| IBIS file stm32f413_f423_ufbga144.ibs
[IBIS ver] 4.2
[File name] stm32f413_f423_ufbga144.ibs
[File Rev] 1.2
[Date]  18-05-2020
[Source] Data Created at STMicroelectronics
[Notes]  File originated from ELDO simulations. rev 1.1: removal of the rising/falling waveform I2C
[Disclaimer]  This information is for modeling purpose only and is
   not guaranted. The information is subject to change without
   notice.
[Copyright] Copyright 2020 STMicroelectronics Inc.
|   Component stm32f413_f423_ufbga144
[Component] stm32f413_f423_ufbga144
[Manufacturer] STMicroelectronics
[Package]
| variable   typ   min   max
R_pkg   0.0   0.0   0.0
L_pkg   0.0H   0.0H   0.0H
C_pkg   0.0F   0.0F   0.0F
[Pin]  signal_name   model_name   R_pin   L_pin   C_pin
A1 PC13-ANTI_TAMP io8p_arwsudq_ft_v33
A10 PA15 io8p_arsudq_ft
A11 PA14 io8p_arsudq_ft
A12 PA13 io8p_arsudq_ft
A2 PE3 io8p_arsudq_ft
A3 PE2 io8p_arsudq_ft
A4 PE1 io8p_arsudq_ft
A5 PE0 io8p_arsudq_ft
A6 PB4 io8p_arsudq_i2cin_ft
A7 PB3 io8p_arsudq_i2c_ft
A8 PD6 io8p_arsudq_ft
A9 PD7 io8p_arsudq_ft
B1 PC14-OSC32_IN io8p_arwsudq_ft
B10 PC11 io8p_arsudq_ft
B11 PC10 io8p_arsudq_ft
B12 PA12 io8usb_vbus_otg_ft
B2 PE4 io8p_arsudq_ft
B3 PE5 io8p_arsudq_ft
B4 PE6 io8p_arsudq_ft
B5 PB9 io8p_arsudq_i2cin_ft
B6 PB5 io8p_ar3wsudq_ft
B7 PG15 io8p_arsudq_ft
B8 PG12 io8p_arsudq_ft
B9 PD5 io8p_arsudq_ft
C1 PC15-OSC32_OUT io8p_arsudq_ft
C10 PC12 io8p_arsudq_ft
C11 VDD_2_USB33 POWER
C12 PA11 io8usb_lsfs_otg_ft
C2 VBAT POWER
C3 PF0 io8p_arsudq_i2cin_ft
C4 PF1 io8p_arsudq_i2cin_ft
C5 PB8 io8p_arsudq_i2cin_ft
C6 PB6 io8p_arsudq_i2cin_ft
C7 PG14 io8p_arsudq_ft
C8 PG11 io8p_arsudq_ft
C9 PD4 io8p_arsudq_ft
D1 PH0-OSC_IN io8p_arsudq_ft
D10 PD1 io8p_arsudq_ft
D11 PA10 io8usb_id_otg_ft
D12 PA9 io8usb_vbus_otg_ft
D2 VSS_5 GND
D3 VDD_5 POWER
D4 PF2 io8p_arsudq_ft
D5 BOOT0 vpp_test_hv
D6 PB7 io8p_arsudq_i2cin_ft
D7 PG13 io8p_arsudq_ft
D8 PG10 io8p_arsudq_ft
D9 PD3 io8p_arsudq_ft
E1 PH1-OSC_OUT io8p_arsudq_ft
E10 PD0 io8p_arsudq_ft
E11 PC9 io8p_arsudq_i2cin_ft
E12 PA8 io8p_arsudq_i2cin_ft
E2 PF3 io8p_arsudq_ft
E3 PF4 io8p_arsudq_ft
E4 PF5 io8p_arsudq_ft
E5 PDR_ON GND
E6 VSS_3 GND
E7 VSS_10 GND
E8 PG9 io8p_arsudq_ft
E9 PD2 io8p_arsudq_ft
F1 NRST ioreset_ft_v33
F10 VDD_9 POWER
F11 PC8 io8p_arsudq_ft
F12 PC7 io8p_arsudq_i2c_ft
F2 PF7 io8p_arsudq_ft
F3 PF6 io8p_arsudq_ft
F4 VDD_4 POWER
F5 VDD_3 POWER
F6 VDD_11 POWER
F7 VDD_10 POWER
F8 VDD_8 POWER
F9 VDD_2_0 POWER
G1 PF10 io8p_arsudq_ft
G10 VSS_2_0 GND
G11 PG8 io8p_arsudq_ft
G12 PC6 io8p_arsudq_i2c_ft
G2 PF9 io8p_arsudq_ft
G3 PF8 io8p_arsudq_ft
G4 VSS_6 GND
G5 VDD_6 POWER
G6 VDD_7 POWER
G7 VDD_1_0 POWER
G8 VSS_8 GND
G9 VCAP2_0 POWER
H1 PC0 io8p_arwsudq_ft_v33
H10 PG7 io8p_arsudq_ft
H11 PG6 io8p_arsudq_ft
H12 PG5 io8p_arsudq_ft
H2 PC1 io8p_arwsudq_ft_v33
H3 PC2 io8p_arwsudq_ft
H4 PC3 io8p_arwsudq_ft
H5 BYPASS_USER GND
H6 VSS_7 GND
H7 VCAP1_0 POWER
H8 PE11 io8p_arsudq_ft
H9 PD11 io8p_arsudq_ft
J1 VSSA GND
J10 PG4 io8p_arsudq_ft
J11 PG3 io8p_arsudq_ft
J12 PG2 io8p_arsudq_ft
J2 PA0-WKUP io8p_arwsudq_ft_v33
J3 PA4 io8p_ar3wsudq_ft
J4 PC4 io8p_arwsudq_ft
J5 PB2 io8p_arwsudq_ft
J6 PG1 io8p_arsudq_ft
J7 PE10 io8p_arsudq_ft
J8 PE12 io8p_arsudq_ft
J9 PD10 io8p_arsudq_ft
K1 VREF- GND
K10 PD13 io8p_arsudq_i2c_ft
K11 PD14 io8p_arsudq_i2c_ft
K12 PD15 io8p_arsudq_i2c_ft
K2 PA1 io8p_arwsudq_ft
K3 PA5 io8p_ar3wsudq_ft
K4 PC5 io8p_arwsudq_ft
K5 PF13 io8p_arsudq_ft
K6 PG0 io8p_arsudq_ft
K7 PE9 io8p_arsudq_ft
K8 PE13 io8p_arsudq_ft
K9 PD9 io8p_arsudq_ft
L1 VREF+ POWER
L10 PD12 io8p_arsudq_i2c_ft
L11 PB14 io8p_arsudq_i2c_ft
L12 PB15 io8p_arsudq_i2c_ft
L2 PA2 io8p_arwsudq_ft
L3 PA6 io8p_ar3wsudq_ft
L4 PB0 io8p_ar3wsudq_ft
L5 PF12 io8p_arsudq_ft
L6 PF15 io8p_arsudq_i2c_ft
L7 PE8 io8p_arsudq_ft
L8 PE14 io8p_arsudq_ft
L9 PD8 io8p_arsudq_ft
M1 VDDA POWER
M10 PB11 io8p_arsudq_i2cin_ft
M11 PB12 io8p_arsudq_ft
M12 PB13 io8p_arsudq_ft
M2 PA3 io8p_arwsudq_ft
M3 PA7 io8p_arwsudq_ft
M4 PB1 io8p_ar3wsudq_ft
M5 PF11 io8p_arsudq_ft
M6 PF14 io8p_arsudq_i2c_ft
M7 PE7 io8p_arsudq_ft
M8 PE15 io8p_ar3wsudq_ft
M9 PB10 io8p_arsudq_i2c_ft
[Model Selector] io8p_ar3wsudq_ft
io8p00_ar3wsudq_ft_pd_lv  "SPEED00 1P8V, PD=40kOhm"
io8p00_ar3wsudq_ft_pu_lv  "SPEED00 1P8V, PU=40kOhm"
io8p00_ar3wsudq_ft_lv  "SPEED00 1P8V"
io8p01_ar3wsudq_ft_pd_lv  "SPEED01 1P8V, PD=40kOhm"
io8p01_ar3wsudq_ft_pu_lv  "SPEED01 1P8V, PU=40kOhm"
io8p01_ar3wsudq_ft_lv  "SPEED01 1P8V"
io8p10_ar3wsudq_ft_pd_lv  "SPEED10 1P8V, PD=40kOhm"
io8p10_ar3wsudq_ft_pu_lv  "SPEED10 1P8V, PU=40kOhm"
io8p10_ar3wsudq_ft_lv  "SPEED10 1P8V"
io8p11_ar3wsudq_ft_pd_lv  "SPEED11 1P8V, PD=40kOhm"
io8p11_ar3wsudq_ft_pu_lv  "SPEED11 1P8V, PU=40kOhm"
io8p11_ar3wsudq_ft_lv  "SPEED11 1P8V"
io8p00_ar3wsudq_ft_pd  "SPEED00, PD=40kOhm"
io8p00_ar3wsudq_ft_pu  "SPEED00, PU=40kOhm"
io8p00_ar3wsudq_ft  "SPEED00"
io8p01_ar3wsudq_ft_pd  "SPEED01, PD=40kOhm"
io8p01_ar3wsudq_ft_pu  "SPEED01, PU=40kOhm"
io8p01_ar3wsudq_ft  "SPEED01"
io8p10_ar3wsudq_ft_pd  "SPEED10, PD=40kOhm"
io8p10_ar3wsudq_ft_pu  "SPEED10, PU=40kOhm"
io8p10_ar3wsudq_ft  "SPEED10"
io8p11_ar3wsudq_ft_pd  "SPEED11, PD=40kOhm"
io8p11_ar3wsudq_ft_pu  "SPEED11, PU=40kOhm"
io8p11_ar3wsudq_ft  "SPEED11"
[Model Selector] io8p_arsudq_ft
io8p00_arsudq_ft_pd_lv  "SPEED00 1P8V, PD=40kOhm"
io8p00_arsudq_ft_pu_lv  "SPEED00 1P8V, PU=40kOhm"
io8p00_arsudq_ft_lv  "SPEED00 1P8V"
io8p01_arsudq_ft_pd_lv  "SPEED01 1P8V, PD=40kOhm"
io8p01_arsudq_ft_pu_lv  "SPEED01 1P8V, PU=40kOhm"
io8p01_arsudq_ft_lv  "SPEED01 1P8V"
io8p10_arsudq_ft_pd_lv  "SPEED10 1P8V, PD=40kOhm"
io8p10_arsudq_ft_pu_lv  "SPEED10 1P8V, PU=40kOhm"
io8p10_arsudq_ft_lv  "SPEED10 1P8V"
io8p11_arsudq_ft_pd_lv  "SPEED11 1P8V, PD=40kOhm"
io8p11_arsudq_ft_pu_lv  "SPEED11 1P8V, PU=40kOhm"
io8p11_arsudq_ft_lv  "SPEED11 1P8V"
io8p00_arsudq_ft_pd  "SPEED00, PD=40kOhm"
io8p00_arsudq_ft_pu  "SPEED00, PU=40kOhm"
io8p00_arsudq_ft  "SPEED00"
io8p01_arsudq_ft_pd  "SPEED01, PD=40kOhm"
io8p01_arsudq_ft_pu  "SPEED01, PU=40kOhm"
io8p01_arsudq_ft  "SPEED01"
io8p10_arsudq_ft_pd  "SPEED10, PD=40kOhm"
io8p10_arsudq_ft_pu  "SPEED10, PU=40kOhm"
io8p10_arsudq_ft  "SPEED10"
io8p11_arsudq_ft_pd  "SPEED11, PD=40kOhm"
io8p11_arsudq_ft_pu  "SPEED11, PU=40kOhm"
io8p11_arsudq_ft  "SPEED11"
[Model Selector] io8p_arsudq_i2c_ft
io8prog_1v8_i2c_pd  "5V Tol GPIO 1.8V range i2c functionality with pull down"
io8prog_1v8_i2c_pu  "5V Tol GPIO 1.8V range i2c functionality with pull up"
io8prog_1v8_i2c  "5V Tol GPIO 1.8V range i2c functionality"
io8prog_3v3_i2c_pd  "5V Tol GPIO 3.3V range i2c functionality with pull down"
io8prog_3v3_i2c_pu  "5V Tol GPIO 3.3V range i2c functionality with pull up"
io8prog_3v3_i2c  "5V Tol GPIO 3.3V range i2c functionality"
io8prog_1v8_pd_00  "5V Tol GPIO 1.8V range with pd speed 00"
io8prog_1v8_pu_00  "5V Tol GPIO 1.8V range with pu speed 00"
io8prog_1v8_00  "5V Tol GPIO 1.8V range speed 00"
io8prog_3v3_pd_00  "5V Tol GPIO 3.3V range with pd speed 00"
io8prog_3v3_pu_00  "5V Tol GPIO 3.3V range with pu speed 00"
io8prog_3v3_00  "5V Tol GPIO 3.3V range speed 00"
io8prog_1v8_pd_01  "5V Tol GPIO 1.8V range with pd speed 01"
io8prog_1v8_pu_01  "5V Tol GPIO 1.8V range with pu speed 01"
io8prog_1v8_01  "5V Tol GPIO 1.8V range speed 01"
io8prog_3v3_pd_01  "5V Tol GPIO 3.3V range with pd speed 01"
io8prog_3v3_pu_01  "5V Tol GPIO 3.3V range with pu speed 01"
io8prog_3v3_01  "5V Tol GPIO 3.3V range speed 01"
io8prog_1v8_pd_10  "5V Tol GPIO 1.8V range with pd speed 10"
io8prog_1v8_pu_10  "5V Tol GPIO 1.8V range with pu speed 10"
io8prog_1v8_10  "5V Tol GPIO 1.8V range speed 10"
io8prog_3v3_pd_10  "5V Tol GPIO 3.3V range with pd speed 10"
io8prog_3v3_pu_10  "5V Tol GPIO 3.3V range with pu speed 10"
io8prog_3v3_10  "5V Tol GPIO 3.3V range speed 10"
io8prog_1v8_pd_11  "5V Tol GPIO 1.8V range with pd speed 11"
io8prog_1v8_pu_11  "5V Tol GPIO 1.8V range with pu speed 11"
io8prog_1v8_11  "5V Tol GPIO 1.8V range speed 11"
io8prog_3v3_pd_11  "5V Tol GPIO 3.3V range with pd speed 11"
io8prog_3v3_pu_11  "5V Tol GPIO 3.3V range with pu speed 11"
io8prog_3v3_11  "5V Tol GPIO 3.3V range speed 11"
[Model Selector] io8p_arsudq_i2cin_ft
io8p00_arsudq_i2cin_ft_pd_lv  "SPEED00 1P8V, PD=40kOhm"
io8p00_arsudq_i2cin_ft_pu_lv  "SPEED00 1P8V, PU=40kOhm"
io8p00_arsudq_i2cin_ft_lv  "SPEED00 1P8V"
io8p01_arsudq_i2cin_ft_pd_lv  "SPEED01 1P8V, PD=40kOhm"
io8p01_arsudq_i2cin_ft_pu_lv  "SPEED01 1P8V, PU=40kOhm"
io8p01_arsudq_i2cin_ft_lv  "SPEED01 1P8V"
io8p10_arsudq_i2cin_ft_pd_lv  "SPEED10 1P8V, PD=40kOhm"
io8p10_arsudq_i2cin_ft_pu_lv  "SPEED10 1P8V, PU=40kOhm"
io8p10_arsudq_i2cin_ft_lv  "SPEED10 1P8V"
io8p11_arsudq_i2cin_ft_pd_lv  "SPEED11 1P8V, PD=40kOhm"
io8p11_arsudq_i2cin_ft_pu_lv  "SPEED11 1P8V, PU=40kOhm"
io8p11_arsudq_i2cin_ft_lv  "SPEED11 1P8V"
io8p00_arsudq_i2cin_ft_pd  "SPEED00, PD=40kOhm"
io8p00_arsudq_i2cin_ft_pu  "SPEED00, PU=40kOhm"
io8p00_arsudq_i2cin_ft  "SPEED00"
io8p01_arsudq_i2cin_ft_pd  "SPEED01, PD=40kOhm"
io8p01_arsudq_i2cin_ft_pu  "SPEED01, PU=40kOhm"
io8p01_arsudq_i2cin_ft  "SPEED01"
io8p10_arsudq_i2cin_ft_pd  "SPEED10, PD=40kOhm"
io8p10_arsudq_i2cin_ft_pu  "SPEED10, PU=40kOhm"
io8p10_arsudq_i2cin_ft  "SPEED10"
io8p11_arsudq_i2cin_ft_pd  "SPEED11, PD=40kOhm"
io8p11_arsudq_i2cin_ft_pu  "SPEED11, PU=40kOhm"
io8p11_arsudq_i2cin_ft  "SPEED11"
[Model Selector] io8p_arwsudq_ft
io8p00_arwsudq_ft_pd_lv  "SPEED00 1P8V, PD=40kOhm"
io8p00_arwsudq_ft_pu_lv  "SPEED00 1P8V, PU=40kOhm"
io8p00_arwsudq_ft_lv  "SPEED00 1P8V"
io8p01_arwsudq_ft_pd_lv  "SPEED01 1P8V, PD=40kOhm"
io8p01_arwsudq_ft_pu_lv  "SPEED01 1P8V, PU=40kOhm"
io8p01_arwsudq_ft_lv  "SPEED01 1P8V"
io8p10_arwsudq_ft_pd_lv  "SPEED10 1P8V, PD=40kOhm"
io8p10_arwsudq_ft_pu_lv  "SPEED10 1P8V, PU=40kOhm"
io8p10_arwsudq_ft_lv  "SPEED10 1P8V"
io8p11_arwsudq_ft_pd_lv  "SPEED11 1P8V, PD=40kOhm"
io8p11_arwsudq_ft_pu_lv  "SPEED11 1P8V, PU=40kOhm"
io8p11_arwsudq_ft_lv  "SPEED11 1P8V"
io8p00_arwsudq_ft_pd  "SPEED00, PD=40kOhm"
io8p00_arwsudq_ft_pu  "SPEED00, PU=40kOhm"
io8p00_arwsudq_ft  "SPEED00"
io8p01_arwsudq_ft_pd  "SPEED01, PD=40kOhm"
io8p01_arwsudq_ft_pu  "SPEED01, PU=40kOhm"
io8p01_arwsudq_ft  "SPEED01"
io8p10_arwsudq_ft_pd  "SPEED10, PD=40kOhm"
io8p10_arwsudq_ft_pu  "SPEED10, PU=40kOhm"
io8p10_arwsudq_ft  "SPEED10"
io8p11_arwsudq_ft_pd  "SPEED11, PD=40kOhm"
io8p11_arwsudq_ft_pu  "SPEED11, PU=40kOhm"
io8p11_arwsudq_ft  "SPEED11"
[Model Selector] io8p_arwsudq_ft_v33
io8p00_arwsudq_ft_v33_pd_lv  "SPEED00 1P8V, PD=40kOhm"
io8p00_arwsudq_ft_v33_pu_lv  "SPEED00 1P8V, PU=40kOhm"
io8p00_arwsudq_ft_v33_lv  "SPEED00 1P8V"
io8p01_arwsudq_ft_v33_pd_lv  "SPEED01 1P8V, PD=40kOhm"
io8p01_arwsudq_ft_v33_pu_lv  "SPEED01 1P8V, PU=40kOhm"
io8p01_arwsudq_ft_v33_lv  "SPEED01 1P8V"
io8p10_arwsudq_ft_v33_pd_lv  "SPEED10 1P8V, PD=40kOhm"
io8p10_arwsudq_ft_v33_pu_lv  "SPEED10 1P8V, PU=40kOhm"
io8p10_arwsudq_ft_v33_lv  "SPEED10 1P8V"
io8p11_arwsudq_ft_v33_pd_lv  "SPEED11 1P8V, PD=40kOhm"
io8p11_arwsudq_ft_v33_pu_lv  "SPEED11 1P8V, PU=40kOhm"
io8p11_arwsudq_ft_v33_lv  "SPEED11 1P8V"
io8p00_arwsudq_ft_v33_pd  "SPEED00, PD=40kOhm"
io8p00_arwsudq_ft_v33_pu  "SPEED00, PU=40kOhm"
io8p00_arwsudq_ft_v33  "SPEED00"
io8p01_arwsudq_ft_v33_pd  "SPEED01, PD=40kOhm"
io8p01_arwsudq_ft_v33_pu  "SPEED01, PU=40kOhm"
io8p01_arwsudq_ft_v33  "SPEED01"
io8p10_arwsudq_ft_v33_pd  "SPEED10, PD=40kOhm"
io8p10_arwsudq_ft_v33_pu  "SPEED10, PU=40kOhm"
io8p10_arwsudq_ft_v33  "SPEED10"
io8p11_arwsudq_ft_v33_pd  "SPEED11, PD=40kOhm"
io8p11_arwsudq_ft_v33_pu  "SPEED11, PU=40kOhm"
io8p11_arwsudq_ft_v33  "SPEED11"
[Model Selector] io8usb_id_otg_ft
io8p00_id_otg_ft_pd_lv  "SPEED00 1P8V, PD=14kOhm"
io8p00_id_otg_ft_pu_lv  "SPEED00 1P8V, PU=14kOhm"
io8p00_id_otg_ft_lv  "SPEED00 1P8V"
io8p01_id_otg_ft_pd_lv  "SPEED01 1P8V, PD=14kOhm"
io8p01_id_otg_ft_pu_lv  "SPEED01 1P8V, PU=14kOhm"
io8p01_id_otg_ft_lv  "SPEED01 1P8V"
io8p10_id_otg_ft_pd_lv  "SPEED10 1P8V, PD=14kOhm"
io8p10_id_otg_ft_pu_lv  "SPEED10 1P8V, PU=14kOhm"
io8p10_id_otg_ft_lv  "SPEED10 1P8V"
io8p11_id_otg_ft_pd_lv  "SPEED11 1P8V, PD=14kOhm"
io8p11_id_otg_ft_pu_lv  "SPEED11 1P8V, PU=14kOhm"
io8p11_id_otg_ft_lv  "SPEED11 1P8V"
io8p00_id_otg_ft_pd  "SPEED00, PD=14kOhm"
io8p00_id_otg_ft_pu  "SPEED00, PU=14kOhm"
io8p00_id_otg_ft  "SPEED00"
io8p01_id_otg_ft_pd  "SPEED01, PD=14kOhm"
io8p01_id_otg_ft_pu  "SPEED01, PU=14kOhm"
io8p01_id_otg_ft  "SPEED01"
io8p10_id_otg_ft_pd  "SPEED10, PD=14kOhm"
io8p10_id_otg_ft_pu  "SPEED10, PU=14kOhm"
io8p10_id_otg_ft  "SPEED10"
io8p11_id_otg_ft_pd  "SPEED11, PD=14kOhm"
io8p11_id_otg_ft_pu  "SPEED11, PU=14kOhm"
io8p11_id_otg_ft  "SPEED11"
[Model Selector] io8usb_lsfs_otg_ft
io8usb_ls_otg_ft_dpdn_pd  "LS USB DP/DN IO + PD=20kOhm"
io8usb_ls_otg_ft_dpdn_pupu2  "LS USB DP/DN IO + PU/PU2=2.2kOhm"
io8usb_ls_otg_ft_dpdn_pu2  "LS USB DP/DN IO + PU2=1.2kOhm"
io8usb_ls_otg_ft_dpdn_pu  "LS USB DP/DN IO + PU=1.2kOhm"
io8usb_ls_otg_ft_dpdn  "LS USB DP/DN IO"
io8usb_fs_otg_ft_dpdn_pd  "HS USB DP/DN IO + PD=20kOhm"
io8usb_fs_otg_ft_dpdn_pupu2  "HS USB DP/DN IO + PU/PU2=2.2kOhm"
io8usb_fs_otg_ft_dpdn_pu2  "HS USB DP/DN IO + PU2=1.2kOhm"
io8usb_fs_otg_ft_dpdn_pu  "HS USB DP/DN IO + PU=1.2kOhm"
io8usb_fs_otg_ft_dpdn  "HS USB DP/DN IO"
io8p00_lsfs_otg_ft_pd_lv  "SPEED00 1P8V, PD=40kOhm"
io8p00_lsfs_otg_ft_pu_lv  "SPEED00 1P8V, PU=40kOhm"
io8p00_lsfs_otg_ft_lv  "SPEED00 1P8V"
io8p01_lsfs_otg_ft_pd_lv  "SPEED01 1P8V, PD=40kOhm"
io8p01_lsfs_otg_ft_pu_lv  "SPEED01 1P8V, PU=40kOhm"
io8p01_lsfs_otg_ft_lv  "SPEED01 1P8V"
io8p10_lsfs_otg_ft_pd_lv  "SPEED10 1P8V, PD=40kOhm"
io8p10_lsfs_otg_ft_pu_lv  "SPEED10 1P8V, PU=40kOhm"
io8p10_lsfs_otg_ft_lv  "SPEED10 1P8V"
io8p11_lsfs_otg_ft_pd_lv  "SPEED11 1P8V, PD=40kOhm"
io8p11_lsfs_otg_ft_pu_lv  "SPEED11 1P8V, PU=40kOhm"
io8p11_lsfs_otg_ft_lv  "SPEED11 1P8V"
io8p00_lsfs_otg_ft_pd  "SPEED00, PD=40kOhm"
io8p00_lsfs_otg_ft_pu  "SPEED00, PU=40kOhm"
io8p00_lsfs_otg_ft  "SPEED00"
io8p01_lsfs_otg_ft_pd  "SPEED01, PD=40kOhm"
io8p01_lsfs_otg_ft_pu  "SPEED01, PU=40kOhm"
io8p01_lsfs_otg_ft  "SPEED01"
io8p10_lsfs_otg_ft_pd  "SPEED10, PD=40kOhm"
io8p10_lsfs_otg_ft_pu  "SPEED10, PU=40kOhm"
io8p10_lsfs_otg_ft  "SPEED10"
io8p11_lsfs_otg_ft_pd  "SPEED11, PD=40kOhm"
io8p11_lsfs_otg_ft_pu  "SPEED11, PU=40kOhm"
io8p11_lsfs_otg_ft  "SPEED11"
[Model Selector] io8usb_vbus_otg_ft
io8psenb_vbus_otg_ft  "VBUS PULSE, SENSE VB"
io8psenab_vbus_otg_ft  "VBUS PULSE, SENSE VA and VB"
io8psena_vbus_otg_ft  "VBUS PULSE, SENSE VA"
io8psen_vbus_otg_ft  "VBUS PULSE"
io8p00_vbus_otg_ft_pd_lv  "SPEED00 1P8V, PD=40kOhm"
io8p00_vbus_otg_ft_pu_lv  "SPEED00 1P8V, PU=40kOhm"
io8p00_vbus_otg_ft_lv  "SPEED00 1P8V"
io8p01_vbus_otg_ft_pd_lv  "SPEED01 1P8V, PD=40kOhm"
io8p01_vbus_otg_ft_pu_lv  "SPEED01 1P8V, PU=40kOhm"
io8p01_vbus_otg_ft_lv  "SPEED01 1P8V"
io8p10_vbus_otg_ft_pd_lv  "SPEED10 1P8V, PD=40kOhm"
io8p10_vbus_otg_ft_pu_lv  "SPEED10 1P8V, PU=40kOhm"
io8p10_vbus_otg_ft_lv  "SPEED10 1P8V"
io8p11_vbus_otg_ft_pd_lv  "SPEED11 1P8V, PD=40kOhm"
io8p11_vbus_otg_ft_pu_lv  "SPEED11 1P8V, PU=40kOhm"
io8p11_vbus_otg_ft_lv  "SPEED11 1P8V"
io8p00_vbus_otg_ft_pd  "SPEED00, PD=40kOhm"
io8p00_vbus_otg_ft_pu  "SPEED00, PU=40kOhm"
io8p00_vbus_otg_ft  "SPEED00"
io8p01_vbus_otg_ft_pd  "SPEED01, PD=40kOhm"
io8p01_vbus_otg_ft_pu  "SPEED01, PU=40kOhm"
io8p01_vbus_otg_ft  "SPEED01"
io8p10_vbus_otg_ft_pd  "SPEED10, PD=40kOhm"
io8p10_vbus_otg_ft_pu  "SPEED10, PU=40kOhm"
io8p10_vbus_otg_ft  "SPEED10"
io8p11_vbus_otg_ft_pd  "SPEED11, PD=40kOhm"
io8p11_vbus_otg_ft_pu  "SPEED11, PU=40kOhm"
io8p11_vbus_otg_ft  "SPEED11"
[Model Selector] ioreset_ft_v33
ioreset_ft_v33_pu_lv  "IORESET 1P8V + PU=40kOhm"
ioreset_ft_v33_nopu_lv  "IORESET 1P8V"
ioreset_ft_v33_pu  "IORESET + PU=40kOhm"
ioreset_ft_v33_nopu  "IORESET"
[Model Selector] vpp_test_hv
vpp_test_hv_2p4  "Input Buffer 1P8V"
vpp_test_hv_3p3  "Input Buffer"
| Models and submodels in the file (242): io8p00_ar3wsudq_ft_pd_lv (I/O), io8p00_ar3wsudq_ft_pu_lv (I/O), io8p00_ar3wsudq_ft_lv (I/O), io8p01_ar3wsudq_ft_pd_lv (I/O), io8p01_ar3wsudq_ft_pu_lv (I/O), io8p01_ar3wsudq_ft_lv (I/O), io8p10_ar3wsudq_ft_pd_lv (I/O), io8p10_ar3wsudq_ft_pu_lv (I/O), io8p10_ar3wsudq_ft_lv (I/O), io8p11_ar3wsudq_ft_pd_lv (I/O), io8p11_ar3wsudq_ft_pu_lv (I/O), io8p11_ar3wsudq_ft_lv (I/O), io8p00_ar3wsudq_ft_pd (I/O), io8p00_ar3wsudq_ft_pu (I/O), io8p00_ar3wsudq_ft (I/O), io8p01_ar3wsudq_ft_pd (I/O), io8p01_ar3wsudq_ft_pu (I/O), io8p01_ar3wsudq_ft (I/O), io8p10_ar3wsudq_ft_pd (I/O), io8p10_ar3wsudq_ft_pu (I/O), io8p10_ar3wsudq_ft (I/O), io8p11_ar3wsudq_ft_pd (I/O), io8p11_ar3wsudq_ft_pu (I/O), io8p11_ar3wsudq_ft (I/O), io8p00_arsudq_ft_pd_lv (I/O), io8p00_arsudq_ft_pu_lv (I/O), io8p00_arsudq_ft_lv (I/O), io8p01_arsudq_ft_pd_lv (I/O), io8p01_arsudq_ft_pu_lv (I/O), io8p01_arsudq_ft_lv (I/O), io8p10_arsudq_ft_pd_lv (I/O), io8p10_arsudq_ft_pu_lv (I/O), io8p10_arsudq_ft_lv (I/O), io8p11_arsudq_ft_pd_lv (I/O), io8p11_arsudq_ft_pu_lv (I/O), io8p11_arsudq_ft_lv (I/O), io8p00_arsudq_ft_pd (I/O), io8p00_arsudq_ft_pu (I/O), io8p00_arsudq_ft (I/O), io8p01_arsudq_ft_pd (I/O), io8p01_arsudq_ft_pu (I/O), io8p01_arsudq_ft (I/O), io8p10_arsudq_ft_pd (I/O), io8p10_arsudq_ft_pu (I/O), io8p10_arsudq_ft (I/O), io8p11_arsudq_ft_pd (I/O), io8p11_arsudq_ft_pu (I/O), io8p11_arsudq_ft (I/O), io8prog_1v8_i2c_pd (I/O), io8prog_1v8_i2c_pu (I/O), io8prog_1v8_i2c (I/O), io8prog_3v3_i2c_pd (I/O), io8prog_3v3_i2c_pu (I/O), io8prog_3v3_i2c (I/O), io8prog_1v8_pd_00 (I/O), io8prog_1v8_pu_00 (I/O), io8prog_1v8_00 (I/O), io8prog_3v3_pd_00 (I/O), io8prog_3v3_pu_00 (I/O), io8prog_3v3_00 (I/O), io8prog_1v8_pd_01 (I/O), io8prog_1v8_pu_01 (I/O), io8prog_1v8_01 (I/O), io8prog_3v3_pd_01 (I/O), io8prog_3v3_pu_01 (I/O), io8prog_3v3_01 (I/O), io8prog_1v8_pd_10 (I/O), io8prog_1v8_pu_10 (I/O), io8prog_1v8_10 (I/O), io8prog_3v3_pd_10 (I/O), io8prog_3v3_pu_10 (I/O), io8prog_3v3_10 (I/O), io8prog_1v8_pd_11 (I/O), io8prog_1v8_pu_11 (I/O), io8prog_1v8_11 (I/O), io8prog_3v3_pd_11 (I/O), io8prog_3v3_pu_11 (I/O), io8prog_3v3_11 (I/O), io8p00_arsudq_i2cin_ft_pd_lv (I/O), io8p00_arsudq_i2cin_ft_pu_lv (I/O)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
